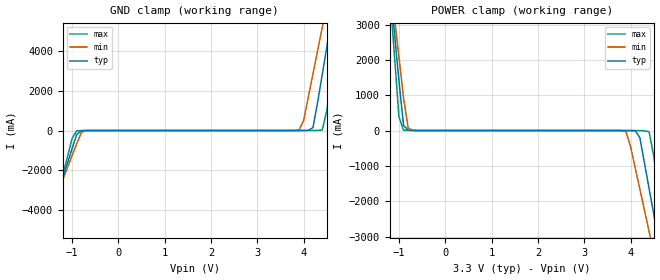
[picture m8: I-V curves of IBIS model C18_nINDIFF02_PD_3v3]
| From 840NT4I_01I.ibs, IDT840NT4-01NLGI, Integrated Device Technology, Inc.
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[Model] C18_nINDIFF02_PD_3v3
Model_type   Input
Polarity   Non-Inverting
Vinl = 0.8V
Vinh = 2.0V
|   typ   min   max
C_comp   2pF   1.5pF   2.5pF
|   typ   min   max
[Voltage range]   3.3V   3.135V   3.465V
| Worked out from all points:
|   GND clamp passes 1 mA (typ) near -0.67 V on its own axis
|   POWER clamp passes 1 mA (typ) near -0.64 V on its own axis
[GND_clamp]
|Voltage   I (typ)   I (min)   I (max)
-3.3V     -17.55A    -15.11A    -21.66A
-1.7V     -5.988A    -5.48A     -6.879A
-1.5V     -4.541A    -4.276A    -5.029A
-900mV    -200.9mA   -666.2mA   -15.02mA
-700mV    -1.318mA   -4.755mA   -1.748mA
3.9V      498.2uA    26.33mA    97.05uA
4.2V      147.2mA    2.842A     2.979mA
4.4V      2.811A     5.169A     26.55mA
4.6V      5.607A     7.497A     2.804A
4.7V      7.005A     8.661A     4.592A
4.8V      8.403A     9.826A     6.38A
6.6V      33.64A     30.86A     38.61A
[Power_clamp]
|Voltage   I (typ)   I (min)   I (max)
-3.3V     33.64A     28.92A     41.58A
-1.2V     4.209A     4.413A     3.966A
-1.1V     2.811A     3.249A     2.179A
-1V       1.414A     2.086A     391.9mA
-900mV    147.2mA    923.7mA    11.43mA
-700mV    1.74mA     4.481mA    2.162mA
3.9V      -290.5uA   -33.14mA   -94.08uA
4.2V      -200.9mA   -1.658A    -2.798mA
4.4V      -1.646A    -2.861A    -35.18mA
4.6V      -3.093A    -4.065A    -1.65A
4.8V      -4.541A    -5.269A    -3.501A
6.6V      -17.55A    -16.1A     -20.14A
